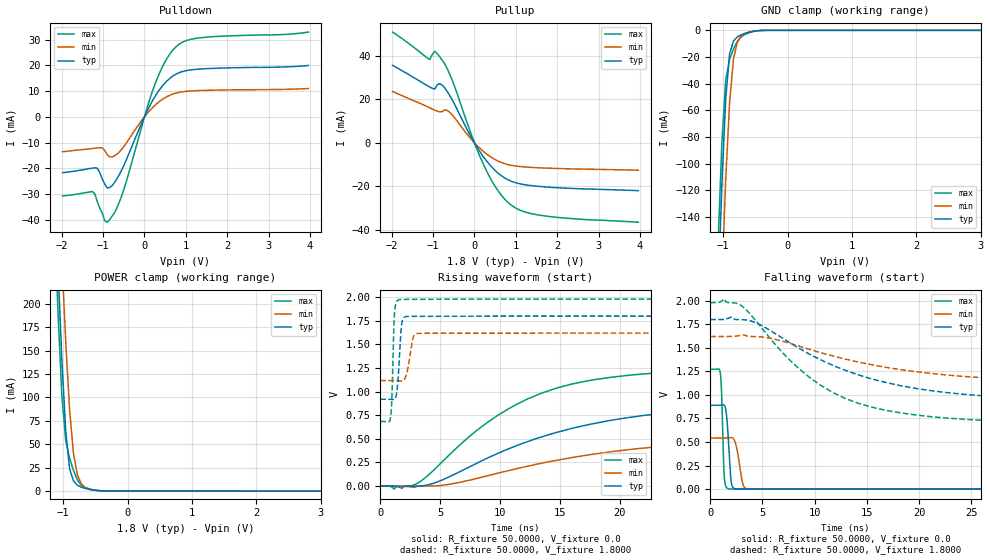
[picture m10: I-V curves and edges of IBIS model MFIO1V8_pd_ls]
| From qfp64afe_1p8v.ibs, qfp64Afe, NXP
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[Model] MFIO1V8_pd_ls
|   Model MFIO1V8_pd_ls
| This model was characterised for following simulation conditions:
| External (pad) voltage:
|   - Typ: 1.8V,   - Min: 1.62V,   - Max: 1.98V
| Library cells for typ/min/max conditions are connected as defined below:
|  IO - External Pad
|  A - Core Input
|  EN - Output Buffer Enable
|  BOOST - vdde
|  EHS - gnd
|  ENZI - vdd
|  EPD - vdd
|  EPUN - vdd
|  ZI - NC
|  ZIF - NC
|  gnd - gnd
|  gnde - gnde
|  vdd - vdd
|  vdde - vdde
| All other pins connected to ground
Model_type I/O
Polarity   Non-Inverting
Enable   Active-Low
Vinl =   0.5400V
Vinh =   1.2600V
Vmeas =  0.9000V
Cref =   0.0F
Rref =   100.0000
Vref =   0.0V
C_comp   1.5958pF   1.5126pF   1.6704pF
|C_comp_pullup   0.7898pF   0.8219pF   0.7460pF
|C_comp_pulldown   0.5931pF   0.6315pF   0.5575pF
[Model Spec]
| variable   typ   min   max
Vinh   0.5400V   0.4860V   0.5940V
Vinl   1.2600V   1.1340V   1.3860V
Vmeas   0.9000V   0.8100V   0.9900V
[Temperature Range]   25.0000   0.1250k   -40.0000
[Voltage Range]   1.8000V   1.6200V   1.9800V
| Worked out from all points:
|   slope of the pulldown table from 0 to 0.27 V, typ, clamps not added: 32.6 ohm
|   slope of the pullup table from 0 to 0.27 V, typ, clamps not added: 34.8 ohm
|   GND clamp passes 1 mA (typ) near -0.56 V on its own axis
|   POWER clamp passes 1 mA (typ) near -0.54 V on its own axis
|   rising waveform, R_fixture 50.0000, V_fixture 0.0: 20-80 % time 13ns typ, 15.7ns min, 9.09ns max; typ from 0 V to 0.89 V
|   rising waveform, R_fixture 50.0000, V_fixture 1.8000: 20-80 % time 250ps typ, 394ps min, 168ps max; typ from 0.92 V to 1.8 V
|   falling waveform, R_fixture 50.0000, V_fixture 0.0: 20-80 % time 296ps typ, 476ps min, 196ps max; typ from 0.89 V to 0 V
|   falling waveform, R_fixture 50.0000, V_fixture 1.8000: 20-80 % time 11.7ns typ, 13.6ns min, 8.55ns max; typ from 1.8 V to 0.92 V
[Pulldown]
|Voltage   I(typ)   I(min)   I(max)
-1.98V    -21.74mA   -13.58mA   -30.76mA
-1.26V    -19.96mA   -12.33mA   -29.04mA
-1.14V    -19.96mA   -12.1mA    -33mA
-960mV    -26.19mA   -13.15mA   -40.44mA
-840mV    -27.51mA   -15.58mA   -39.92mA
-540mV    -20.34mA   -12.41mA   -30.2mA
60mV      2.086mA    1.197mA    3.341mA
300mV     9.043mA    5.145mA    14.58mA
540mV     13.88mA    7.813mA    22.59mA
840mV     17.16mA    9.517mA    28.23mA
1.44V     18.67mA    10.27mA    30.87mA
3.96V     19.95mA    10.98mA    32.93mA
[Pullup]
|Voltage   I(typ)   I(min)   I(max)
-1.98V    35.7mA     23.68mA    51.03mA
-1.08V    25.71mA    16.17mA    38.42mA
-960mV    24.81mA    15.04mA    42.18mA
-840mV    27.29mA    14.27mA    39.65mA
-720mV    25.36mA    15.21mA    36.42mA
-540mV    19.88mA    12.94mA    28.95mA
-60mV     2.001mA    1.263mA    3.041mA
240mV     -7.02mA    -4.333mA   -10.88mA
600mV     -14.41mA   -8.644mA   -22.88mA
900mV     -17.74mA   -10.36mA   -28.83mA
1.74V     -20.33mA   -11.62mA   -33.75mA
3.96V     -22mA      -12.58mA   -36.53mA
[GND_clamp]
|Voltage   I(typ)   I(min)   I(max)
-1.98V    -1.781A    -1.801A    -1.77A
-1.08V    -200.1mA   -270.2mA   -162.2mA
-1.02V    -116mA     -186.2mA   -84.49mA
-960mV    -51.26mA   -111.8mA   -37.36mA
-900mV    -17.65mA   -54.44mA   -21.7mA
-840mV    -8.02mA    -21.7mA    -14.08mA
-780mV    -4.924mA   -8.964mA   -8.313mA
-720mV    -3.338mA   -4.442mA   -4.753mA
-600mV    -1.403mA   -1.338mA   -1.896mA
-480mV    -330.4uA   -347.3uA   -423.3uA
-360mV    -26.82uA   -39.45uA   -30.02uA
3.96V     0A         0A         0A
[POWER_clamp]
|Voltage   I(typ)   I(min)   I(max)
-1.98V    2.119A     2.147A     2.105A
-1.14V    349.2mA    450mA      300.6mA
-1.08V    239.1mA    345.9mA    191.2mA
-1.02V    140.4mA    247.8mA    101.7mA
-960mV    64.08mA    159.3mA    53.89mA
-900mV    23.59mA    87.23mA    35.11mA
-840mV    10.79mA    40.2mA     22.07mA
-780mV    6.218mA    17.5mA     11.92mA
-720mV    4.013mA    7.752mA    6.009mA
-600mV    1.739mA    1.846mA    2.368mA
-360mV    67.5uA     96.07uA    73.34uA
3.96V     0A         0A         0A
[Ramp]
| variable   typ   min   max
dV/dt_r  0.5338/12.9648n   0.3251/15.7125n   0.7629/9.0945n
dV/dt_f  0.5279/11.7476n   0.3013/13.6114n   0.7770/8.5474n
R_load = 50.0000
[Rising Waveform]
R_fixture= 50.0000
V_fixture= 0.0
V_fixture_min= 0.0
V_fixture_max= 0.0
|time   V(typ)   V(min)   V(max)
0s        1.134nV    103.8nV    53.92pV
1.143ns   -48.43uV   18.14uV    -32.5mV
3.218ns   -124.7uV   -1.778mV   38.38mV
8.04ns    241.9mV    80.85mV    588.1mV
12.33ns   472.2mV    211.6mV    924.4mV
15.97ns   610mV      301.6mV    1.079V
21.23ns   734.6mV    393.2mV    1.179V
28.9ns    822.7mV    469.2mV    1.234V
40.83ns   869.5mV    518mV      1.262V
100ns     889.6mV    541.8mV    1.272V
[Rising Waveform]
R_fixture= 50.0000
V_fixture= 1.8000
V_fixture_min= 1.6200
V_fixture_max= 1.9800
|time   V(typ)   V(min)   V(max)
0s        919.5mV    1.117V     684.3mV
848.4ps   919.7mV    1.117V     717.4mV
970.5ps   917.8mV    1.117V     936mV
1.192ns   916mV      1.117V     1.838V
1.419ns   1.034V     1.116V     1.963V
1.644ns   1.476V     1.113V     1.974V
1.927ns   1.777V     1.117V     1.976V
2.742ns   1.797V     1.572V     1.976V
3.289ns   1.797V     1.617V     1.976V
100ns     1.799V     1.619V     1.979V
[Falling Waveform]
R_fixture= 50.0000
V_fixture= 0.0
V_fixture_min= 0.0
V_fixture_max= 0.0
|time   V(typ)   V(min)   V(max)
0s        889.7mV    541.9mV    1.272V
954.8ps   889.9mV    542mV      1.235V
1.081ns   891.9mV    541.9mV    1.036V
1.348ns   889.9mV    541.7mV    123.7mV
1.583ns   758.1mV    542.8mV    13.13mV
1.815ns   361.3mV    545.9mV    2.908mV
2.135ns   24.48mV    543.6mV    1.242mV
3.157ns   889.4uV    41.34mV    1.38mV
3.783ns   1.039mV    1.515mV    1.077mV
100ns     20.55nV    161.7nV    7.279nV
[Falling Waveform]
R_fixture= 50.0000
V_fixture= 1.8000
V_fixture_min= 1.6200
V_fixture_max= 1.9800
|time   V(typ)   V(min)   V(max)
0s        1.799V     1.619V     1.979V
1.308ns   1.8V       1.619V     2.017V
3.053ns   1.798V     1.634V     1.941V
4.706ns   1.748V     1.617V     1.74V
7.856ns   1.537V     1.539V     1.344V
11.74ns   1.314V     1.413V     1.025V
15.17ns   1.179V     1.326V     878.9mV
20.52ns   1.055V     1.236V     776.1mV
39.53ns   936.6mV    1.132V     693.8mV
100ns     919.5mV    1.117V     684.3mV
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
